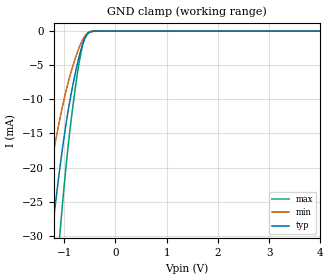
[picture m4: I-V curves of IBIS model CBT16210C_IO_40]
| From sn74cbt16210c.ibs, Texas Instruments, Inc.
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[Model]   CBT16210C_IO_40
Model_type  Terminator
| variable   typ   min   max
C_comp   5.80pF   4.32pF   8.55pF
| C_tri-state   5.80pF   4.32pF   8.55pF
[Temperature Range]   40   100   -40
| Ambient temperature   25   85   -40
[Voltage range]   4   4   4
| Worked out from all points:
|   GND clamp passes 1 mA (typ) near -0.59 V on its own axis
[GND Clamp]
| CBT16210C_IO_40
|   Voltage   I(typ)   I(min)   I(max)
-4V       -296.1mA   -216.4mA   -384.1mA
-1.455V   -45.62mA   -29.44mA   -67.39mA
-1.24V    -29.99mA   -19.2mA    -44.73mA
-1.205V   -27.66mA   -17.7mA    -41.27mA
-1.08V    -19.94mA   -12.78mA   -29.59mA
-910mV    -11.21mA   -7.246mA   -16.12mA
-755mV    -5.273mA   -3.395mA   -6.972mA
-695mV    -3.395mA   -2.188mA   -4.131mA
-635mV    -1.864mA   -1.225mA   -1.947mA
-580mV    -875.1uA   -611.9uA   -715.7uA
-515mV    -258.9uA   -210.2uA   -139.2uA
4V        419.1pA    1.535nA    95.06pA
